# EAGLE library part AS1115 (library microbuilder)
AS1115 - 64 LED (8 * 7-Segment) LED Driver VDD: 2.7-5.5V Digikey: AS1115-BSSTCT-ND
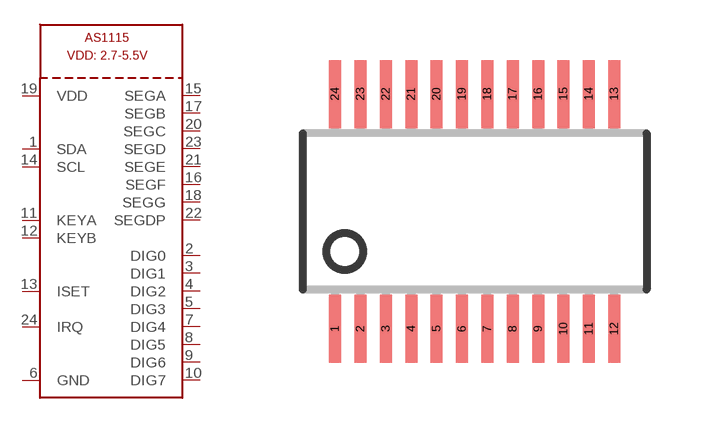
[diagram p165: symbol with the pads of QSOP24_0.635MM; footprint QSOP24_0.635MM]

Designator prefix U

## AS1115  [QSOP24_0.635MM]
1  SDA
2  DIG0
3  DIG1
4  DIG2
5  DIG3
6  GND
7  DIG4
8  DIG5
9  DIG6
10  DIG7
11  KEYA
12  KEYB
13  ISET
14  SCL
15  SEGA
16  SEGF
17  SEGB
18  SEGG
19  VDD
20  SEGC
21  SEGE
22  SEGDP
23  SEGD
24  IRQ

## Footprint QSOP24_0.635MM (pad centres in mm)
smd 0.3 x 1.7: 1 -3.493,-2.935; 2 -2.857,-2.935; 3 -2.223,-2.935; 4 -1.587,-2.935; 5 -0.953,-2.935; 6 -0.318,-2.935; 7 0.318,-2.935; 8 0.953,-2.935; 9 1.587,-2.935; 10 2.223,-2.935; 11 2.857,-2.935; 12 3.493,-2.935; 13 3.493,2.935; 14 2.857,2.935; 15 2.223,2.935; 16 1.587,2.935; 17 0.953,2.935; 18 0.318,2.935; 19 -0.318,2.935; 20 -0.953,2.935; 21 -1.587,2.935; 22 -2.223,2.935; 23 -2.857,2.935; 24 -3.493,2.935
